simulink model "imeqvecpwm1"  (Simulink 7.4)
settings: Solver=ode45  StartTime=0.0  StopTime=2  MaxStep=5e-6  RelTol=1e-4  AbsTol=1e-6
libraries: simulink x1

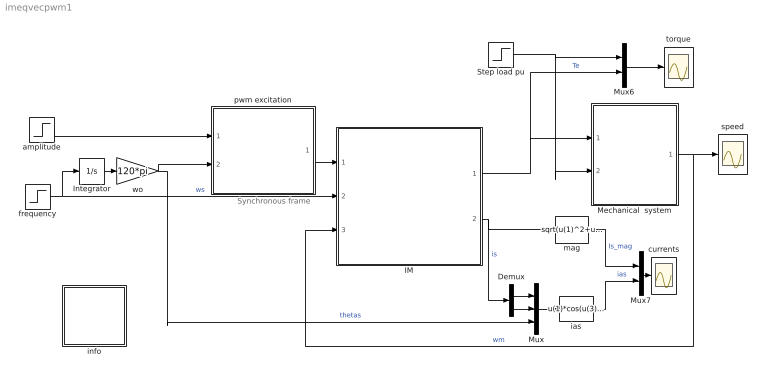
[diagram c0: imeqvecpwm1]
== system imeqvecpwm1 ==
  note: Synchronous frame
  Demux : Demux  Outputs=2
  IM : Subsystem  mask{Rs=0.01, Rr=0.02, Lsl=0.10, Lrl=0.10, Lm=4.5, wo=2*pi*60}
      mask prompts: Rs "Stator resistance [pu]"; Rr "Rotor resistance [pu]"; Lsl "Stator leakage inductance [pu]"; Lrl "Rotor leakage inductance [pu]"; Lm "Magnetizing inductance [pu]"; wo "Base frequency [rad/s]"
      mask help: Induction machine dynamic model in the synchronous frame
  Integrator : Integrator
  Mechanical  system : Subsystem  mask{H=0.3, Bm=1e-5}
      mask prompts: H "Inertia constant [s]"; Bm "Torque-speed coefficient"
  Mux : Mux  Inputs=3
  Mux6 : Mux  Inputs=2
  Mux7 : Mux  Inputs=2
  Step load pu : Step  Time=1.7  SampleTime=0
  amplitude : Step  Time=1.4  Before=1  After=5/6  SampleTime=0
  currents : Scope
  frequency : Step  Time=1.4  Before=1  After=5/6  SampleTime=0
  ias : Fcn  Expr=u(1)*cos(u(3))-u(2)*sin(u(3))
  info : Subsystem
  mag : Fcn  Expr=sqrt(u(1)^2+u(2)^2)
  pwm excitation : Subsystem
  speed : Scope
  torque : Scope
  wo : Gain  Gain=120*pi  ParameterDataType=sfix(16)  ParameterScaling=2^0  OutDataType=sfix(16)  OutScaling=2^0
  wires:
  amplitude/1 -> pwm excitation/1(vs)
  Integrator/1 -> wo/1
  Mux/1 -> ias/1
  ias/1 -> Mux7/2  "ias"
  mag/1 -> Mux7/1  "Is_mag"
  Mux7/1 -> currents/1
  Demux/1 -> Mux/1
  Demux/2 -> Mux/2
  IM/2(is) -> mag/1, Demux/1  "is"
  Mux6/1 -> torque/1
  Step load pu/1 -> Mux6/1, Mechanical  system/2(Tl)
  IM/1(Te) -> Mux6/2, Mechanical  system/1(Te)  "Te"
  wo/1 -> pwm excitation/2(thetas), Mux/3  "thetas"
  Mechanical  system/1(wm) -> IM/3(wm), speed/1  "wm"
  pwm excitation/1(dq) -> IM/1(vs)
  frequency/1 -> IM/2(Iwk), Integrator/1  "ws"

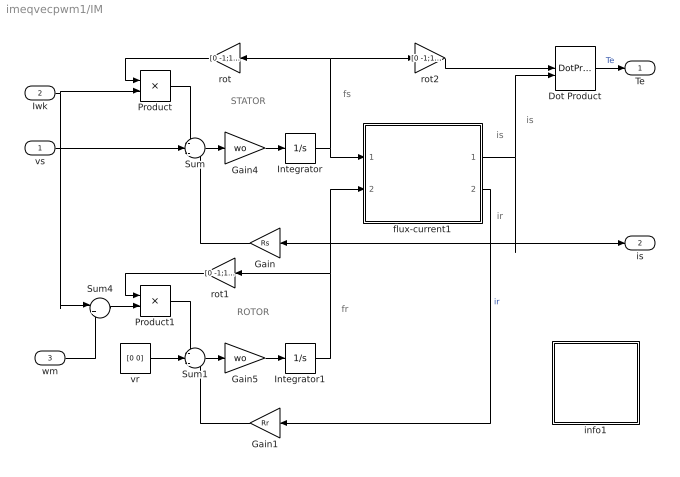
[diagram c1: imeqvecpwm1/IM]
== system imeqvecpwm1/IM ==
  note: ROTOR
  note: STATOR
  note: fs
  note: fr
  note: is
  note: is
  note: ir
  vs : Inport  OutDataType=sfix(16)  OutScaling=2^0
  Iwk : Inport  Port=2  OutDataType=sfix(16)  OutScaling=2^0
  wm : Inport  Port=3  OutDataType=sfix(16)  OutScaling=2^0
  Dot Product : DotProduct  OutDataType=fixdt(1, 16)  OutScaling=2^-10
  Gain : Gain  Gain=Rs  ParameterDataType=sfix(16)  ParameterScaling=2^0  OutDataType=sfix(16)  OutScaling=2^0
  Gain1 : Gain  Gain=Rr  ParameterDataType=sfix(16)  ParameterScaling=2^0  OutDataType=sfix(16)  OutScaling=2^0
  Gain4 : Gain  Gain=wo  ParameterDataType=sfix(16)  ParameterScaling=2^0  OutDataType=sfix(16)  OutScaling=2^0
  Gain5 : Gain  Gain=wo  ParameterDataType=sfix(16)  ParameterScaling=2^0  OutDataType=sfix(16)  OutScaling=2^0
  Integrator : Integrator  InitialCondition=[0 0]
  Integrator1 : Integrator  InitialCondition=[0 0]
  Product : Product  OutDataType=sfix(16)  OutScaling=2^0
  Product1 : Product  OutDataType=sfix(16)  OutScaling=2^0
  Sum : Sum  Inputs=-+-  OutDataType=sfix(16)  OutScaling=2^0
  Sum1 : Sum  Inputs=-+-  OutDataType=sfix(16)  OutScaling=2^0
  Sum4 : Sum  Inputs=|+-  OutDataType=sfix(16)  OutScaling=2^0
  flux-current1 : Subsystem
  info1 : Subsystem
  rot : Gain  Gain=[0 -1;1 0]  Multiplication=Matrix(K*u)  ParameterDataType=sfix(16)  ParameterScaling=2^0  OutDataType=sfix(16)  OutScaling=2^0
  rot1 : Gain  Gain=[0 -1;1 0]  Multiplication=Matrix(K*u)  ParameterDataType=sfix(16)  ParameterScaling=2^0  OutDataType=sfix(16)  OutScaling=2^0
  rot2 : Gain  Gain=[0 -1;1 0]  Multiplication=Matrix(K*u)  ParameterDataType=sfix(16)  ParameterScaling=2^0  OutDataType=sfix(16)  OutScaling=2^0
  vr : Constant  Value=[0 0]  OutDataType=sfix(16)  OutScaling=2^0
  Te : Outport
  is : Outport  Port=2
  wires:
  Gain/1 -> Sum/3
  vr/1 -> Sum1/2
  Gain1/1 -> Sum1/3
  flux-current1/2(ir) -> Gain1/1  "ir"
  Integrator/1 -> flux-current1/1(fs), rot/1, rot2/1
  Integrator1/1 -> flux-current1/2(fr), rot1/1
  Product1/1 -> Sum1/1
  rot1/1 -> Product1/1
  Product/1 -> Sum/1
  rot/1 -> Product/1
  rot2/1 -> Dot Product/1
  Sum4/1 -> Product1/2
  Sum/1 -> Gain4/1
  Gain4/1 -> Integrator/1
  Sum1/1 -> Gain5/1
  Gain5/1 -> Integrator1/1
  flux-current1/1(is) -> Gain/1, is/1, Dot Product/2
  Dot Product/1 -> Te/1  "Te"
  vs/1 -> Sum/2
  Iwk/1 -> Product/2, Sum4/1
  wm/1 -> Sum4/2

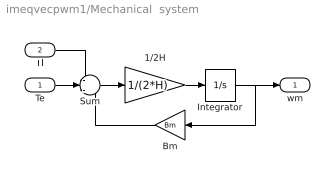
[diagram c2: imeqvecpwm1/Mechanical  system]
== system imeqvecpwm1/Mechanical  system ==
  Te : Inport  OutDataType=sfix(16)  OutScaling=2^0
  Tl : Inport  Port=2  OutDataType=sfix(16)  OutScaling=2^0
  1/2H : Gain  Gain=1/(2*H)  ParameterDataType=sfix(16)  ParameterScaling=2^0  OutDataType=sfix(16)  OutScaling=2^0
  Bm : Gain  Gain=Bm  ParameterDataType=sfix(16)  ParameterScaling=2^0  OutDataType=sfix(16)  OutScaling=2^0
  Integrator : Integrator
  Sum : Sum  Inputs=-+-  OutDataType=sfix(16)  OutScaling=2^0
  wm : Outport
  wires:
  1/2H/1 -> Integrator/1
  Sum/1 -> 1/2H/1
  Bm/1 -> Sum/3
  Integrator/1 -> Bm/1, wm/1
  Te/1 -> Sum/2
  Tl/1 -> Sum/1

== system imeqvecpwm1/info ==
  note: This demo deals with the open-loop operation of an induction motor that is excited by means of a sinusoidal PWM inverter and reproduces the conditions encountered in the simulation entitled 'im3frames.mdl' which involves a pure 3-phase sinusoidal excitation. Except for the appearance of the high frequency components, the transient characteristics are almost iden- tical . The filtering action of inertia produces the same speed versus time curves. The main difference in the two simulations is that the presence a triangular carrier at 5KHz necessitates the use of a very small integration time step of a few microseconds.
  note: Starting of an Induction Motor at no Load under Sinusoidal PWM Excitation

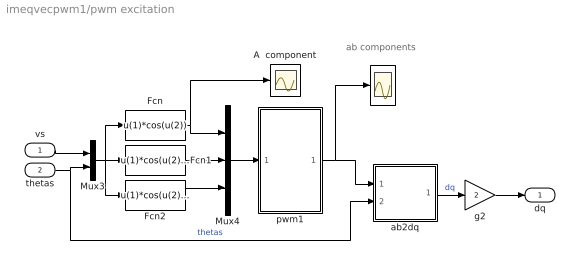
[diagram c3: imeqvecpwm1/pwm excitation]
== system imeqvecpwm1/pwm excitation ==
  note: ab components
  vs : Inport  OutDataType=sfix(16)  OutScaling=2^0
  thetas : Inport  Port=2  OutDataType=sfix(16)  OutScaling=2^0
  " " : Scope
  A  component : Scope
  Fcn : Fcn  Expr=u(1)*cos(u(2))
  Fcn1 : Fcn  Expr=u(1)*cos(u(2)-2*pi/3)
  Fcn2 : Fcn  Expr=u(1)*cos(u(2)+2*pi/3)
  Mux3 : Mux  Inputs=2
  Mux4 : Mux  Inputs=3
  ab2dq : Subsystem
  g2 : Gain  Gain=2  ParameterDataType=sfix(16)  ParameterScaling=2^0  OutDataType=sfix(16)  OutScaling=2^0
  pwm1 : Subsystem
  dq : Outport
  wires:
  Mux3/1 -> Fcn/1, Fcn1/1, Fcn2/1
  thetas/1 -> Mux3/2, ab2dq/2(thetak)  "thetas"
  vs/1 -> Mux3/1
  ab2dq/1(dq) -> g2/1  "dq"
  g2/1 -> dq/1
  Mux4/1 -> pwm1/1(ABC)
  Fcn/1 -> A  component/1, Mux4/1
  Fcn1/1 -> Mux4/2
  Fcn2/1 -> Mux4/3
  pwm1/1(ab) -> ab2dq/1(ab), " "/1

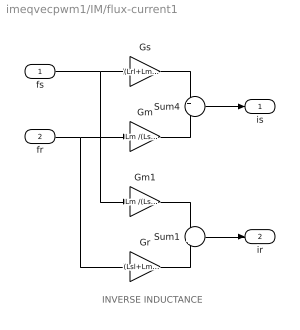
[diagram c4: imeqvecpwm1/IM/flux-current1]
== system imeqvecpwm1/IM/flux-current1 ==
  note: INVERSE INDUCTANCE
  fs : Inport  OutDataType=sfix(16)  OutScaling=2^0
  fr : Inport  Port=2  OutDataType=sfix(16)  OutScaling=2^0
  Gm : Gain  Gain=Lm /(Lsl*Lrl+Lsl*Lm+Lrl*Lm)  ParameterDataType=sfix(16)  ParameterScaling=2^0  OutDataType=sfix(16)  OutScaling=2^0
  Gm1 : Gain  Gain=Lm /(Lsl*Lrl+Lsl*Lm+Lrl*Lm)  ParameterDataType=sfix(16)  ParameterScaling=2^0  OutDataType=sfix(16)  OutScaling=2^0
  Gr : Gain  Gain=(Lsl+Lm )/(Lsl*Lrl+Lsl*Lm+Lrl*Lm)  ParameterDataType=sfix(16)  ParameterScaling=2^0  OutDataType=sfix(16)  OutScaling=2^0
  Gs : Gain  Gain=(Lrl+Lm) /(Lsl*Lrl+Lsl*Lm+Lrl*Lm)  ParameterDataType=sfix(16)  ParameterScaling=2^0  OutDataType=sfix(16)  OutScaling=2^0
  Sum1 : Sum  Inputs=-+  OutDataType=sfix(16)  OutScaling=2^0
  Sum4 : Sum  Inputs=+-  OutDataType=sfix(16)  OutScaling=2^0
  is : Outport
  ir : Outport  Port=2
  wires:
  fs/1 -> Gs/1, Gm1/1
  Gs/1 -> Sum4/1
  fr/1 -> Gm/1, Gr/1
  Gm/1 -> Sum4/2
  Sum4/1 -> is/1
  Gm1/1 -> Sum1/1
  Gr/1 -> Sum1/2
  Sum1/1 -> ir/1

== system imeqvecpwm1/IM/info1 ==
  note: This demonstration illustrates the dynamics of a synchronous generator, initially at no load, following a three-phase short circuit at the terminals.
  note: Synchronous machine transients under shortcircuit

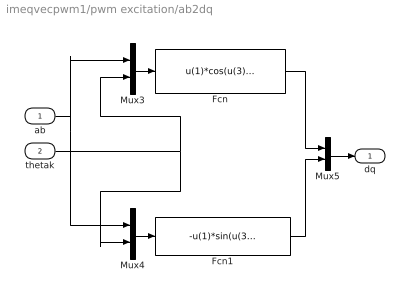
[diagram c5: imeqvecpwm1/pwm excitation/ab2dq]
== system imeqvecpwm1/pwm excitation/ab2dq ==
  ab : Inport  OutDataType=sfix(16)  OutScaling=2^0
  thetak : Inport  Port=2  OutDataType=sfix(16)  OutScaling=2^0
  Fcn : Fcn  Expr=u(1)*cos(u(3))+u(2)*sin(u(3))
  Fcn1 : Fcn  Expr=-u(1)*sin(u(3))+u(2)*cos(u(3))
  Mux3 : Mux  Inputs=2
  Mux4 : Mux  Inputs=2
  Mux5 : Mux  Inputs=2
  dq : Outport
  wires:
  Mux3/1 -> Fcn/1
  Mux4/1 -> Fcn1/1
  ab/1 -> Mux3/1, Mux4/1
  thetak/1 -> Mux3/2, Mux4/2
  Fcn1/1 -> Mux5/2
  Fcn/1 -> Mux5/1
  Mux5/1 -> dq/1

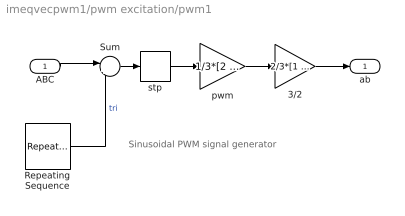
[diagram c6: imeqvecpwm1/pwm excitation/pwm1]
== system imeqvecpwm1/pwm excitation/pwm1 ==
  note: Sinusoidal PWM signal generator
  ABC : Inport  OutDataType=sfix(16)  OutScaling=2^0
  3/2 : Gain  Gain=2/3*[1 -0.5 -0.5;0 sqrt(3)/2 -sqrt(3)/2]  Multiplication=Matrix(K*u)  ParameterDataType=sfix(16)  ParameterScaling=2^0  OutDataType=sfix(16)  OutScaling=2^0
  Repeating Sequence : simulink/Sources/Repeating Sequence  SystemSampleTime=-1  rep_seq_t="[0  0.5/5000 1/5000]"  rep_seq_y=[1 -1 1]
  Sum : Sum  Inputs=|+-  OutDataType=sfix(16)  OutScaling=2^0
  pwm : Gain  Gain=1/3*[2 -1 -1;-1 2 -1;-1 -1 2]  Multiplication=Matrix(K*u)  ParameterDataType=sfix(16)  ParameterScaling=2^0  OutDataType=sfix(16)  OutScaling=2^0
  stp : Relay  OutDataType=sfix(16)  OutScaling=2^0
  ab : Outport
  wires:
  Sum/1 -> stp/1
  Repeating Sequence/1 -> Sum/2  "tri"
  stp/1 -> pwm/1
  pwm/1 -> 3/2/1
  3/2/1 -> ab/1
  ABC/1 -> Sum/1
